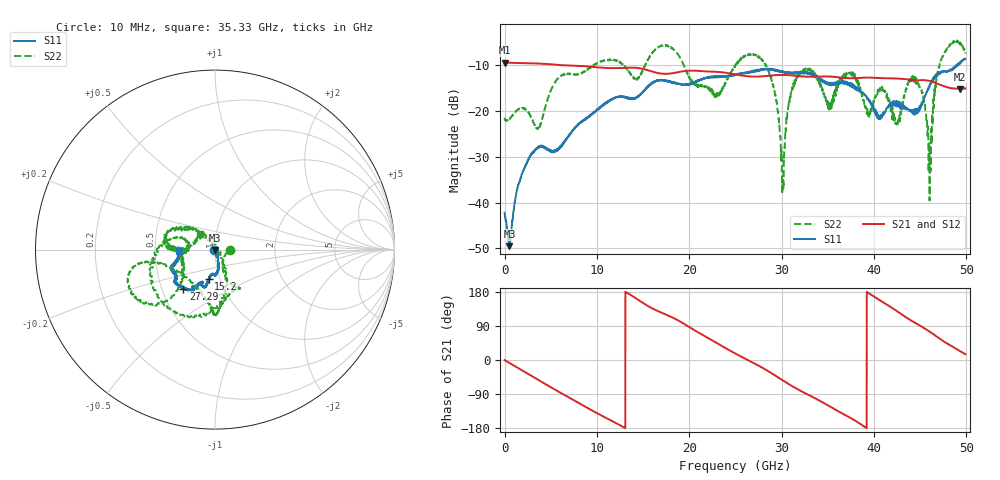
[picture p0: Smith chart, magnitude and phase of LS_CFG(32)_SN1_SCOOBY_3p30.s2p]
!Keysight Technologies,N5245B,MY58422026,A.13.80.08
!Date: Thursday, March 19, 2020 23:36:48
!Correction: S11(Full 2 Port(1,2))
!S21(Full 2 Port(1,2))
!S12(Full 2 Port(1,2))
!S22(Full 2 Port(1,2))
!S2P File: Measurements: S11, S21, S12, S22:
# Hz S DB R 50.0
!freq dBS11 angS11 dBS21 angS21 dBS12 angS12 dBS22 angS22
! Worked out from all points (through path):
!   4991 points, 10 MHz to 49.91 GHz, reference 50 ohm
!   highest |S21| = -9.41 dB at 10 MHz (marker M1); lowest = -15.1 dB at 49.34 GHz (marker M2)
!   group delay of S21, straight-line fit = 38.7 ps
!   lowest |S11| = -49.5 dB at 530 MHz (marker M3), VSWR 1.01, Z = 49.7 - j0.215 ohm
!   |S11| at or under -10 dB: start of sweep to 48.9 GHz; 48.92734 GHz to 48.99762 GHz (70.28 MHz wide, 0.144 % of centre); 49.06614 GHz to 49.09396 GHz (27.82 MHz wide, 0.0567 % of centre)
!   |S22| runs from -39.6 to -4.6 dB; largest |S21 - S12| = 0.003
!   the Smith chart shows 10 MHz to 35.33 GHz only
!   S11 on the Smith chart (normalised r, x): 10 MHz: 0.99, -0.01; 15.2 GHz: 0.88, -0.30; 27.29 GHz: 0.64, -0.30; 35.33 GHz: 0.67, -0.01
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1e7  -42.19 -158.5  -9.41 -0.3  -9.39 -0.3  -21.48 0.3
5.3e8  -49.53 -139.6  -9.45 -7.7  -9.44 -7.7  -21.68 -10.3
2.8e9  -29.71 -58.1  -9.58 -40.0  -9.57 -40.0  -21.02 -0.3
8.33e9  -22.50 -76.6  -10.14 -117.5  -10.14 -117.5  -11.71 -70.9
1.52e10  -15.47 -102.3  -10.91 147.4  -10.90 147.5  -10.13 -166.5
1.665e10  -13.33 -105.8  -11.70 128.6  -11.69 128.7  -6.06 -163.8
2.289e10  -12.65 -116.4  -11.43 46.2  -11.43 46.3  -16.97 174.1
2.496e10  -12.13 -120.3  -11.96 17.6  -11.95 17.7  -10.27 179.1
2.729e10  -11.04 -129.0  -12.47 -12.0  -12.46 -11.8  -7.87 -113.2
2.911e10  -10.87 -141.2  -12.18 -37.9  -12.18 -37.8  -14.32 -70.2
3.014e10  -11.49 -145.0  -12.14 -53.8  -12.15 -53.6  -35.32 42.5
3.116e10  -11.64 -147.6  -12.23 -69.1  -12.24 -68.8  -14.80 142.9
3.328e10  -11.90 -160.4  -12.49 -96.8  -12.49 -96.4  -11.32 176.5
3.533e10  -14.03 -177.7  -12.48 -123.8  -12.43 -123.5  -18.33 132.9
3.734e10  -14.36 168.6  -12.81 -151.5  -12.72 -151.6  -11.73 137.8
4.16e10  -18.77 101.0  -12.86 143.2  -12.88 143.1  -17.76 32.1
4.253e10  -18.12 93.8  -12.89 128.4  -12.91 128.3  -23.11 -9.2
4.457e10  -19.84 45.2  -13.26 96.8  -13.29 96.7  -13.11 -13.1
4.603e10  -14.50 5.5  -13.40 74.9  -13.42 75.0  -39.56 -7.4
4.712e10  -11.51 9.0  -14.21 56.4  -14.22 56.5  -9.68 -96.6
4.934e10  -9.54 -19.5  -15.14 23.3  -15.16 23.5  -4.94 -34.6
4.991e10  -8.60 -17.0  -15.05 15.3  -15.07 15.2  -7.19 -21.7
